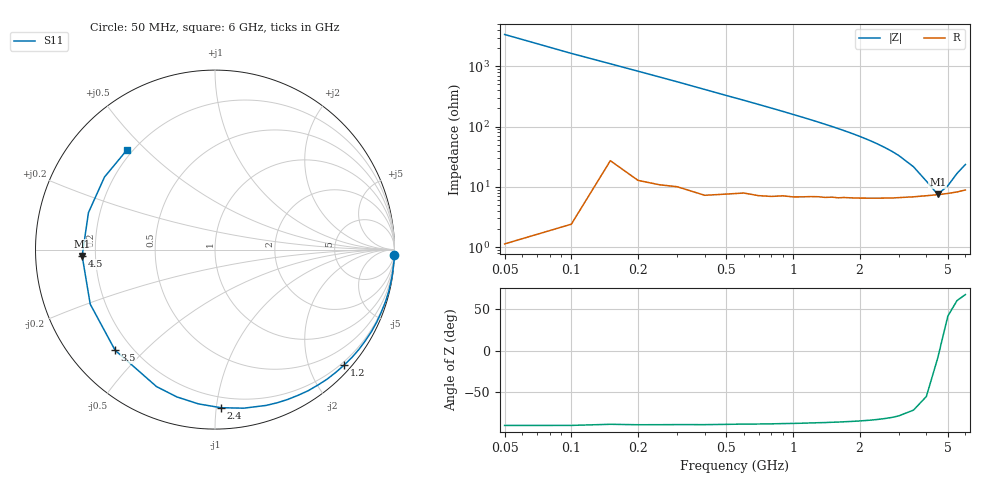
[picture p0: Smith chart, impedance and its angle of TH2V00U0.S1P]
! SIEMENS Discrete & RF Semiconductors
! BAS70
! Si Schottky Diode in SOT23
! VR = 2 V
! S-Parameters:  February  1997
# GHz  S  MA  R  50
!  f  S11
! GHz  MAG  ANG
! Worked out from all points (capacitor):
!   34 points, 50 MHz to 6 GHz, reference 50 ohm
!   read as one part to ground: C = 963 fF near 50 MHz
!   lowest |Z| = 7.53 ohm at 4.5 GHz (marker M1)
!   series resonance near 4.571 GHz, so ESL is about 1.3 nH
!   S11 on the Smith chart (normalised r, x): 50 MHz: 0, -67; 1.2 GHz: 0.14, -2.61; 2.4 GHz: 0.13, -1.03; 3.5 GHz: 0.14, -0.41; 4.5 GHz: 0.15, -0.02; 6 GHz: 0.18, +0.44
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0.05  1 -1.7
0.1  0.9999 -3.5
0.25  0.9976 -8.6
0.4  0.9958 -13.8
0.5  0.9931 -17.3
0.6  0.9898 -20.7
0.7  0.9875 -24.2
0.8  0.9841 -27.7
1  0.9758 -34.8
1.1  0.9709 -38.3
1.2  0.9651 -41.9
1.4  0.9545 -49.2
1.5  0.9477 -52.8
1.6  0.9421 -56.6
1.8  0.928 -64.1
1.9  0.9211 -67.9
2  0.9137 -71.8
2.2  0.898 -79.7
2.4  0.8817 -87.8
2.6  0.8646 -96.1
2.8  0.8478 -104.5
3  0.8299 -113.1
3.5  0.7901 -134.8
4  0.7587 -156.4
4.5  0.7409 -177.3
5  0.7346 163.7
5.5  0.7365 146.7
6  0.7405 131.7
